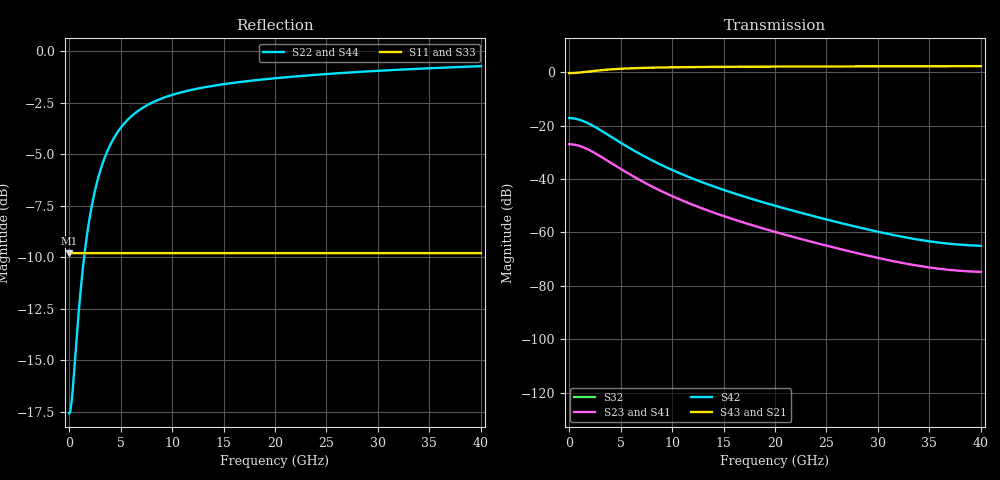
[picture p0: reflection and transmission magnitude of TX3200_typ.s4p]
# hz S ri R 50
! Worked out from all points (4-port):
!   20000 points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, 2 MHz to 40 GHz, reference 50 ohm
!   strongest paths, dB at 2 MHz, 10 GHz, 20 GHz, 30 GHz, 40 GHz:
!     S43: -0.4, 1.8, 2.1, 2.2, 2.2
!     S21: -0.4, 1.8, 2.1, 2.2, 2.2
!     S42: -17.2, -36.6, -50.0, -59.8, -65.0
!     S23: -27.0, -46.4, -59.8, -69.6, -74.8
!     S41: -27.0, -46.4, -59.8, -69.6, -74.8
!     S32: -, -, -, -, -
!   lowest |S11| = -9.8 dB at 2 MHz (marker M1), VSWR 1.96, Z = 97.9 + j0 ohm
!   |S11| at or under -10 dB: nowhere
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2000000  0.3236 0  0 0  0 0  0 0
         0.9572 0.00017  0.1321 -0.000527  -0.0448 5.26e-05  0.1384 -0.000163
         0 0  0 0  0.3236 0  0 0
         -0.0448 5.26e-05  0.1384 -0.000163  0.9602 0.000167  0.1229 -0.000516
2.372e9  0.3236 0  0 0  0 0  0 0
         1.042 0.1368  -0.1307 -0.4226  -0.0113 0.0295  0.035 -0.091
         0 0  0 0  0.3236 0  0 0
         -0.0113 0.0295  0.035 -0.091  1.043 0.1356  -0.1328 -0.4188
6.214e9  0.3236 0  0 0  0 0  0 0
         1.174 0.1457  -0.5383 -0.4501  0.00705 0.00876  -0.0218 -0.0271
         0 0  0 0  0.3236 0  0 0
         0.00705 0.00876  -0.0218 -0.0271  1.175 0.1466  -0.541 -0.4528
1.257e10  0.3236 0  0 0  0 0  0 0
          1.241 0.1068  -0.7433 -0.3299  0.0029 0.00071  -0.00895 -0.00219
          0 0  0 0  0.3236 0  0 0
          0.0029 0.000711  -0.00895 -0.0022  1.243 0.1068  -0.7506 -0.3301
2.1162e10  0.3236 0  0 0  0 0  0 0
           1.268 0.0812  -0.829 -0.2508  0.000865 -0.000182  -0.00267 0.000563
           0 0  0 0  0.3236 0  0 0
           0.000865 -0.000181  -0.00267 0.00056  1.27 0.0799  -0.8346 -0.247
3.245e10  0.3236 0  0 0  0 0  0 0
          1.285 0.0648  -0.8817 -0.2001  0.000153 -0.000218  -0.000472 0.000672
          0 0  0 0  0.3236 0  0 0
          0.000153 -0.000217  -0.000474 0.000671  1.286 0.0634  -0.8838 -0.1959
4e10  0.3236 0  0 0  0 0  0 0
      1.292 0.0575  -0.9037 -0.1775  -2.64e-05 -0.00018  8.17e-05 0.000556
      0 0  0 0  0.3236 0  0 0
      -2.59e-05 -0.000179  8e-05 0.000555  1.293 0.0564  -0.9045 -0.1742
